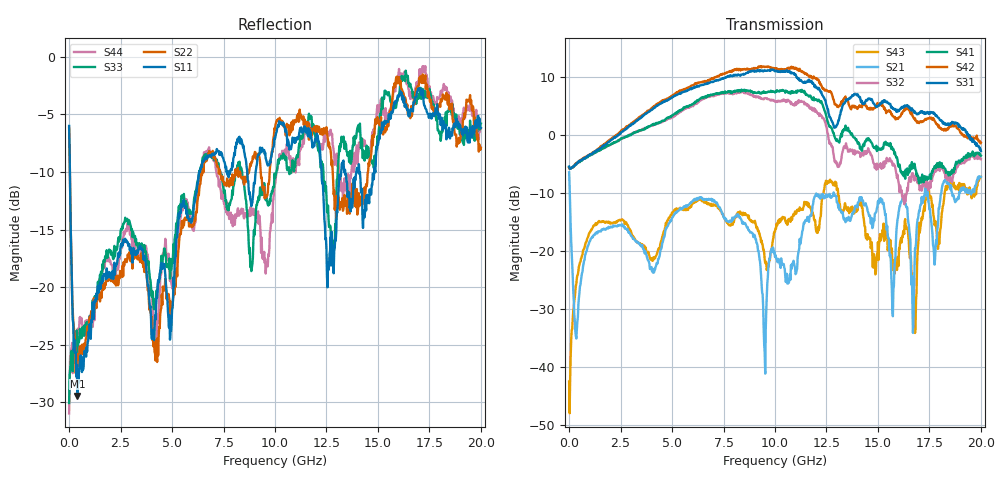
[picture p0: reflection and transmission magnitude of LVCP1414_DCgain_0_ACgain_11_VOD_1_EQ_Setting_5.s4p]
!Agilent Technologies,N5230A,MY46400459,A.07.50.48
!Agilent N5230A: A.07.50.48
!Date: Tuesday, April 17, 2012 18:31:17
!Correction: S11(Full 4 Port(1,2,3,4))
!S12(Full 4 Port(1,2,3,4))
!S13(Full 4 Port(1,2,3,4))
!S14(Full 4 Port(1,2,3,4))
!S21(Full 4 Port(1,2,3,4))
!S22(Full 4 Port(1,2,3,4))
!S23(Full 4 Port(1,2,3,4))
!S24(Full 4 Port(1,2,3,4))
!S31(Full 4 Port(1,2,3,4))
!S32(Full 4 Port(1,2,3,4))
!S33(Full 4 Port(1,2,3,4))
!S34(Full 4 Port(1,2,3,4))
!S41(Full 4 Port(1,2,3,4))
!S42(Full 4 Port(1,2,3,4))
!S43(Full 4 Port(1,2,3,4))
!S44(Full 4 Port(1,2,3,4))
!S4P File: Measurements: <S11,S12,S13,S14>,
!<S21,S22,S23,S24>,
!<S31,S32,S33,S34>,
!<S41,S42,S43,S44>:
# Hz S  dB  R 50
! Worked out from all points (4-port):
!   801 points, 300 kHz to 20 GHz, reference 50 ohm
!   strongest paths, dB at 300 kHz, 5 GHz, 10 GHz, 15 GHz, 20 GHz:
!     S31: -5.5, 6.5, 11.0, 5.0, -2.8
!     S42: -5.7, 6.8, 11.4, 5.3, -1.4
!     S41: -5.6, 3.4, 7.3, -2.1, -3.6
!     S32: -5.6, 3.0, 5.8, -5.9, -4.2
!     S21: -6.5, -14.3, -21.1, -11.5, -7.3
!     S43: -42.6, -13.4, -16.7, -18.5, -7.3
!   lowest |S11| = -29.4 dB at 400.3 MHz (marker M1), VSWR 1.07, Z = 53.2 + j1.46 ohm
!   |S11| at or under -10 dB: 37.55 MHz to 6.32 GHz (6.283 GHz wide, 198 % of centre); 12.26 GHz to 13.21 GHz (953.2 MHz wide, 7.48 % of centre); 14.09 GHz to 14.82 GHz (720.7 MHz wide, 4.99 % of centre)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
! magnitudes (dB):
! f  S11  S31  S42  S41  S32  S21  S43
! 300 kHz  -6.0  -5.5  -5.7  -5.6  -5.6  -6.5  -42.6
! 400.3 MHz  -29.4  -4.8  -4.8  -4.9  -4.9  -32.2  -24.2
! 9.975 GHz  -7.0  11.1  11.4  7.4  5.8  -20.1  -16.7
! 12.75 GHz  -15.2  2.4  7.1  1.2  -2.0  -10.8  -8.1
! 16.78 GHz  -3.9  4.1  2.7  -5.0  -7.9  -23.0  -30.0
! 17.4 GHz  -4.9  3.9  2.8  -7.7  -8.5  -9.8  -10.3
! 20 GHz  -6.2  -2.8  -1.4  -3.6  -4.2  -7.3  -7.3
